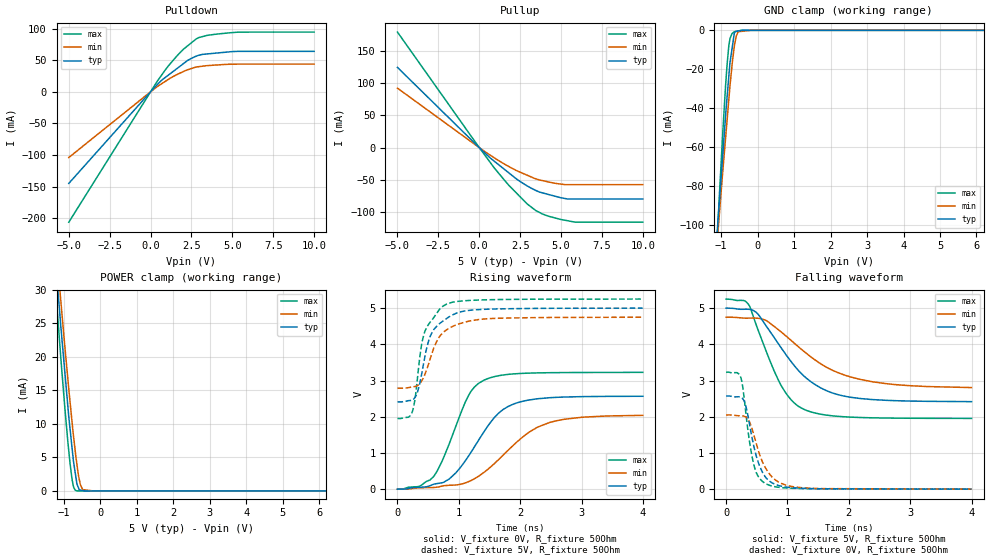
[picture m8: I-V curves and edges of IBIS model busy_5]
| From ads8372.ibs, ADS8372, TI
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|   busy_5 Model
[Model]   busy_5
Model_type   3-state
Polarity   Non-Inverting
Vmeas = 2.5
Vref = 2.5
Cref = 10pF
Rref = 50
|   typ   min   max
|   (nom PVT)   (fast PVT)   (slow PVT)
|C_comp from frequency sweep method (F=1MHz)
|C_comp   2.602e-12   2.596e-12   2.649e-12
|ON state : BUFFER OUTPUT TURNED HIGH
|C_comp   2.602e-12   2.596e-12   2.649e-12
|OFF state: BUFFER IN HIGH IMPEDANCE
|C_comp   2.720e-12   2.612e-12   2.807e-12
|C_comp from LC tank measurement(L=1nH)
|Resonant Frequency(Hz)   6.320e+09   6.380e+09   6.200e+09
|C_comp   6.348e-13   6.229e-13   6.596e-13
|ON state : BUFFER OUTPUT TURNED HIGH
|Resonant Frequency(Hz)   6.320e+09   6.380e+09   6.200e+09
|C_comp   6.348e-13   6.229e-13   6.596e-13
|OFF state: BUFFER IN HIGH IMPEDANCE
|Resonant Frequency(Hz)   6.310e+09   6.400e+09   6.190e+09
C_comp   6.368e-13   6.190e-13   6.617e-13
| Where nom  PVT is Nominal Process, 5V, 35C
|   Fast PVT is Strong Process,  5.25V, -40C
|   Slow PVT is Weak Process,   4.75V, 95C
[Voltage Range]   5   4.75   5.25
|Ambient Temperature   25   85   -40
|Junction Temperature
[Temperature Range]   35   95   -40
[Pullup Reference]   5   4.75   5.25
[Pulldown Reference]   0   0   0
[Power Clamp Reference]   5   4.75   5.25
[GND Clamp Reference]   0   0   0
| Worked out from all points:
|   slope of the pulldown table from 0 to 0.75 V, typ, clamps not added: 38 ohm
|   slope of the pullup table from 0 to 0.75 V, typ, clamps not added: 42.3 ohm
|   GND clamp passes 1 mA (typ) near -0.62 V on its own axis
|   POWER clamp passes 1 mA (typ) near -0.64 V on its own axis
|   falling waveform, V_fixture 5V, R_fixture 50Ohm: 20-80 % time 748ps typ, 977ps min, 512ps max; typ from 5 V to 2.42 V
|   rising waveform, V_fixture 0V, R_fixture 50Ohm: 20-80 % time 638ps typ, 838ps min, 467ps max; typ from 0 V to 2.56 V
|   rising waveform, V_fixture 5V, R_fixture 50Ohm: 20-80 % time 265ps typ, 314ps min, 228ps max; typ from 2.41 V to 5 V
|   falling waveform, V_fixture 0V, R_fixture 50Ohm: 20-80 % time 227ps typ, 284ps min, 168ps max; typ from 2.57 V to 0.002 V
[Pulldown]
|   Voltage   I(typ)   I(min)   I(max)
-5V       -144.9mA   -103.9mA   -206.2mA
425.3mV   11.75mA    8.409mA    17.37mA
924mV     23.18mA    16.95mA    35.51mA
1.596V    36.42mA    27.07mA    56.31mA
2.011V    44.59mA    32.13mA    67.4mA
2.27V     49.69mA    34.93mA    72.81mA
2.793V    56.42mA    39.22mA    83.73mA
3.46V     59.87mA    41.37mA    89.24mA
5.318V    63.92mA    43.76mA    94.26mA
10V       63.98mA    43.79mA    94.45mA
[GND Clamp]
|   Voltage   I(typ)   I(min)   I(max)
-5V       -1.317A    -1.15A     -1.875A
-1.088V   -97.97mA   -103.5mA   -99.09mA
-1.045V   -86.82mA   -93.3mA    -83.33mA
-955.5mV  -63.76mA   -72.34mA   -52.55mA
-834.7mV  -33.62mA   -45.54mA   -17mA
-792.7mV  -24.22mA   -36.22mA   -8.58mA
-756mV    -16.39mA   -28.15mA   -4.121mA
-640.5mV  -1.642mA   -8.441mA   -729.4uA
-584.3mV  -563.8uA   -2.825mA   -508.2uA
-532mV    -390.4uA   -718.3uA   -302.8uA
-190mV    0A         -32.43nA   -2.902uA
10V       0A         0A         0A
[Pullup]
|   Voltage   I(typ)   I(min)   I(max)
-5V       124.5mA    92.27mA    179.4mA
115.6fV   -79.82pA   -98.94pA   -72.32pA
924mV     -21.25mA   -15.91mA   -31.72mA
1.822V    -39.47mA   -29.55mA   -58.86mA
2.27V     -48.57mA   -35.64mA   -70.41mA
2.94V     -59.62mA   -42.98mA   -87.67mA
3.465V    -66.64mA   -48.5mA    -97.83mA
4.058V    -71.6mA    -52.31mA   -104.9mA
5.405V    -79.77mA   -57.54mA   -113.6mA
5.87V     -79.77mA   -57.54mA   -115.8mA
10V       -79.77mA   -57.54mA   -115.8mA
[POWER Clamp]
|   Voltage   I(typ)   I(min)   I(max)
-5V       555.6mA    444.8mA    819.5mA
-1.306V   39.53mA    42.72mA    35.96mA
-1.088V   24.91mA    28.69mA    20.27mA
-971.2mV  17.69mA    21.51mA    12.38mA
-829.5mV  9.28mA     13.29mA    4.118mA
-771.8mV  6.287mA    10.14mA    1.651mA
-687.7mV  2.707mA    5.963mA    93.45uA
-640mV    1.014mA    3.922mA    9.836uA
-546.3mV  125.6uA    929.3uA    1.201uA
-484.5mV  66.71uA    197.5uA    1.066uA
-190mV    0A         22.35nA    418.1nA
10V       0A         0A         0A
[Ramp]
R_load = 50
|   typ   min   max
dV/dt_r   1.53909/6.3631e-10   1.22282/8.30702e-10   1.93489/4.65884e-10
dV/dt_f   1.54923/7.47558e-10   1.16617/9.76263e-10   1.977/5.12193e-10
[Falling Waveform]
V_fixture = 5V
V_fixture_min = 4.75V
V_fixture_max = 5.25V
R_fixture = 50Ohm
|   Time   V(typ)   V(min)   V(max)
0s        5V         4.75V      5.25V
362ps     4.969V     4.723V     5.109V
518ps     4.837V     4.72V      4.409V
866ps     3.98V      4.384V     2.959V
1.054ns   3.534V     4.115V     2.479V
1.246ns   3.16V      3.836V     2.223V
1.69ns    2.683V     3.319V     2.034V
2.194ns   2.503V     3.029V     1.979V
2.992ns   2.434V     2.858V     1.959V
3.998ns   2.418V     2.806V     1.955V
[Rising Waveform]
V_fixture = 0V
V_fixture_min = 0V
V_fixture_max = 0V
R_fixture = 50Ohm
|   Time   V(typ)   V(min)   V(max)
0s        1.729nV    3.388nV    1.523nV
354ps     51.69mV    37.14mV    78.35mV
586ps     134.3mV    45.86mV    342.7mV
844ps     281.7mV    108.1mV    1.254V
1.15ns    893.4mV    201.1mV    2.559V
1.41ns    1.586V     463.7mV    3.009V
1.798ns   2.278V     1.066V     3.168V
2.146ns   2.463V     1.575V     3.204V
2.474ns   2.524V     1.838V     3.216V
3.998ns   2.565V     2.038V     3.225V
[Rising Waveform]
V_fixture = 5V
V_fixture_min = 4.75V
V_fixture_max = 5.25V
R_fixture = 50Ohm
|   Time   V(typ)   V(min)   V(max)
0s        2.412V     2.79V      1.953V
234ps     2.456V     2.82V      2.107V
282ps     2.523V     2.833V     2.444V
328ps     2.692V     2.863V     3.097V
384ps     3.082V     2.959V     3.898V
438ps     3.576V     3.129V     4.311V
552ps     4.288V     3.695V     4.653V
798ps     4.708V     4.397V     5.107V
1.432ns   4.967V     4.702V     5.228V
3.998ns   4.998V     4.748V     5.249V
[Falling Waveform]
V_fixture = 0V
V_fixture_min = 0V
V_fixture_max = 0V
R_fixture = 50Ohm
|   Time   V(typ)   V(min)   V(max)
0s        2.57V      2.048V     3.227V
238ps     2.543V     2.028V     3.089V
316ps     2.331V     1.997V     2.182V
378ps     1.824V     1.871V     1.344V
448ps     1.215V     1.522V     705.1mV
534ps     692.4mV    1.018V     324mV
660ps     294.8mV    538mV      140mV
860ps     99.11mV    192mV      52.96mV
1.208ns   27.3mV     45.18mV    18.38mV
3.998ns   2.059mV    2.042mV    1.4mV
